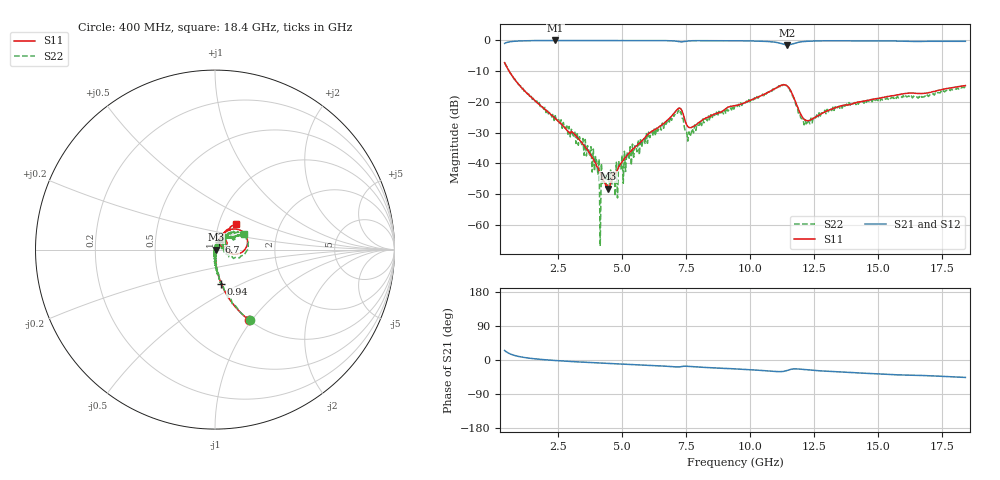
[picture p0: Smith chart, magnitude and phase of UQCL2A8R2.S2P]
! AVX Corporation
! Date:  10/27/06
! Part No:  UQCL2A8R2
! Description:  Ultra Low ESR Microwave capacitors
! Mounting Orientation:  Horizontal
# GHZ S DB R 50
! Freq  |S11|  S11 Ph  |S21|  S21 Ph  |S12|  S12 Ph  |S22|  S22 Ph
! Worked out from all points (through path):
!   401 points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, 400 MHz to 18.4 GHz, reference 50 ohm
!   highest |S21| = -0.04 dB at 2.38 GHz (marker M1); lowest = -1.5 dB at 11.43 GHz (marker M2)
!   group delay of S21, straight-line fit = 7.96 ps
!   lowest |S11| = -48.2 dB at 4.45 GHz (marker M3), VSWR 1.01, Z = 50.4 - j0.0394 ohm
!   |S11| at or under -10 dB: 574.5 MHz to end of sweep
!   |S22| runs from -66.9 to -7.2 dB; largest |S21 - S12| = 0.0056
!   S11 on the Smith chart (normalised r, x): 400 MHz: 1.00, -0.96; 940 MHz: 0.99, -0.39; 6.7 GHz: 1.04, +0.09; 18.4 GHz: 1.21, +0.35
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0.4  -7.25 -64.3  -0.98 25.0  -0.96 24.9  -7.16 -63.4
0.94  -14.23 -79.7  -0.21 9.4  -0.18 9.4  -14.26 -77.9
2.38  -25.40 -86.8  -0.04 -1.4  -0.03 -1.4  -24.48 -92.6
3.415  -33.16 -85.9  -0.05 -5.6  -0.03 -5.6  -33.90 -107.3
4  -41.03 -69.8  -0.05 -7.6  -0.03 -7.7  -39.40 -66.0
4.045  -41.21 -70.0  -0.05 -7.7  -0.03 -7.8  -43.70 -143.0
4.135  -43.23 -61.3  -0.04 -8.0  -0.03 -8.1  -66.89 145.5
4.225  -44.90 -51.4  -0.05 -8.3  -0.03 -8.4  -46.52 -12.2
4.27  -45.58 -45.9  -0.05 -8.5  -0.03 -8.6  -43.29 -147.0
4.45  -48.16 -5.7  -0.05 -9.1  -0.04 -9.2  -44.95 74.6
4.72  -43.23 34.4  -0.05 -10.0  -0.04 -10.1  -50.65 -33.8
5.17  -37.46 57.3  -0.06 -11.4  -0.05 -11.5  -36.36 54.4
6.43  -28.13 65.3  -0.08 -15.4  -0.08 -15.6  -28.59 59.4
6.7  -26.41 64.8  -0.10 -16.4  -0.11 -16.6  -27.32 69.8
7.195  -22.08 43.5  -0.39 -18.4  -0.40 -18.6  -22.64 37.1
7.6  -28.30 32.3  -0.20 -16.9  -0.21 -17.1  -29.73 34.0
9.4  -21.25 61.5  -0.14 -23.4  -0.16 -23.7  -21.18 50.6
11.425  -14.75 9.8  -1.48 -27.9  -1.48 -27.9  -14.70 1.0
12.01  -24.63 -1.4  -0.46 -24.6  -0.47 -24.7  -25.45 -15.8
12.415  -25.55 37.2  -0.23 -27.1  -0.24 -27.1  -26.82 34.1
15.43  -18.16 59.5  -0.20 -38.1  -0.22 -38.0  -18.60 36.3
18.4  -14.71 50.6  -0.32 -46.0  -0.35 -45.9  -14.86 28.1
